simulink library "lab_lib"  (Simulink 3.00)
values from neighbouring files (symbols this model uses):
  h = 0.01    [design.m]    (also in initfra.m; initlab1.m; tst.m)
  R = [1 80 1600]    [tst.m]
  S = [3200]    [tst.m]
  T = 2*pi/w    [fra.m]
libraries: lab_lib x3, cstblocks x1

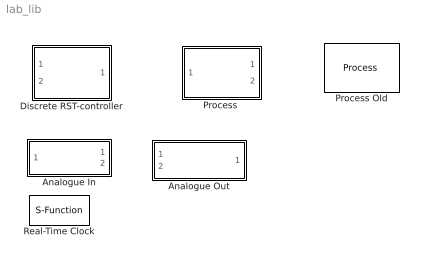
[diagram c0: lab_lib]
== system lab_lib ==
  Analogue In : Subsystem  mask(AnalogueIOBlock){AIno=}
      mask prompts: AIno "Input port number"
      mask help: Analogue input block for use on PC running Linux.
  Analogue Out : Subsystem  mask(AnalogueIOBlock){AOno=}
      mask prompts: AOno "Output port number"
      mask help: Analogue output block for use on PC running Linux
  Discrete RST-controller : Subsystem  mask(ControllerMaskBlock){R=R, S=S, T=T, h=h}
      mask prompts: R "R-polynomial"; S "S-polynomial"; T "T-polynomial"; h "Sample period"
      mask help: Discrete RST-controller (forward shift) R(q)u = -S(q)y + T(q)y_ref
  "Process " : Subsystem  mask(SISO Process){AOno=0, AIno=0, h=h}
      mask prompts: AOno "AO connection"; AIno "AI connection"; h "Sample Period"
      mask help: Process communication block. For use with Linux on PC with I/O.
  Process Old : lab_lib/Process   AOno=0  AIno=0  h=h
  Real-Time Clock : S-Function  FunctionName=timer  Parameters=h  PortCounts=[]  SFunctionModules=''

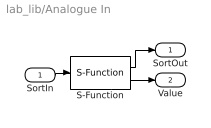
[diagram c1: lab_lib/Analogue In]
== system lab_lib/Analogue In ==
  SortIn : Inport  Port=1  PortWidth=-1  SampleTime=-1  DataType=auto
  S-Function : S-Function  FunctionName=analogin  Parameters=AIno  PortCounts=[]  SFunctionModules=''
  SortOut : Outport  Port=1  InitialOutput=0
  Value : Outport  Port=2  InitialOutput=0
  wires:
  S-Function/1 -> SortOut/1
  SortIn/1 -> S-Function/1
  S-Function/2 -> Value/1

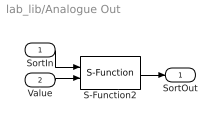
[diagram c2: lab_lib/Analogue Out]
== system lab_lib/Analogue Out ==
  SortIn : Inport  Port=1  PortWidth=-1  SampleTime=-1  DataType=auto
  Value : Inport  Port=2  PortWidth=-1  SampleTime=-1  DataType=auto
  S-Function2 : S-Function  FunctionName=analogout  Parameters=AOno  PortCounts=[]  SFunctionModules=''
  SortOut : Outport  Port=1  InitialOutput=0
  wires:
  SortIn/1 -> S-Function2/1
  S-Function2/1 -> SortOut/1
  Value/1 -> S-Function2/2

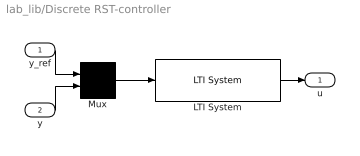
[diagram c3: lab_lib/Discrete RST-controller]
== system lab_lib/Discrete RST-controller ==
  y_ref : Inport  Port=1  PortWidth=-1  SampleTime=-1  DataType=auto
  y : Inport  Port=2  PortWidth=-1  SampleTime=-1  DataType=auto
  LTI System : cstblocks/LTI System  sys=ss(tf({T,-S},{R,R},h))  IC=[0]
  Mux : Mux  Inputs=2
  u : Outport  Port=1  InitialOutput=0
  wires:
  Mux/1 -> LTI System/1
  y_ref/1 -> Mux/1
  LTI System/1 -> u/1
  y/1 -> Mux/2

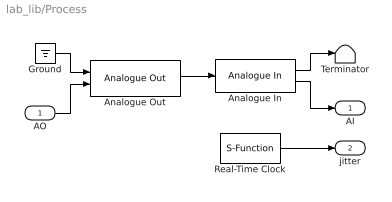
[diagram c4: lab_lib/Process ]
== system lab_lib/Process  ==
  AO : Inport  Port=1  PortWidth=-1  SampleTime=-1  DataType=auto
  Analogue In : lab_lib/Analogue In  AIno=AIno
  Analogue Out : lab_lib/Analogue Out  AOno=AOno
  Ground : Ground
  Real-Time Clock : S-Function  FunctionName=timer  Parameters=h  PortCounts=[]  SFunctionModules=''
  Terminator : Terminator
  AI : Outport  Port=1  InitialOutput=0
  jitter : Outport  Port=2
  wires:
  AO/1 -> Analogue Out/2
  Ground/1 -> Analogue Out/1
  Real-Time Clock/1 -> jitter/1
  Analogue In/2 -> AI/1
  Analogue In/1 -> Terminator/1
  Analogue Out/1 -> Analogue In/1
